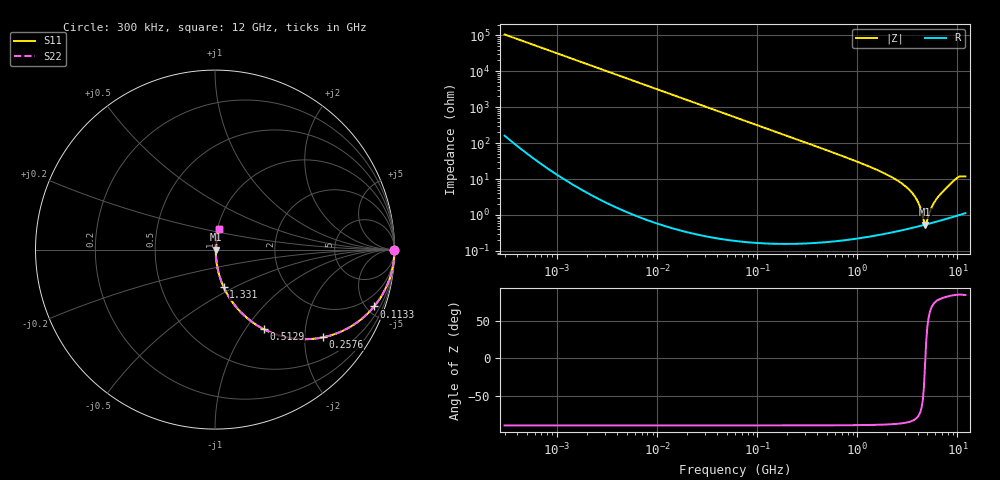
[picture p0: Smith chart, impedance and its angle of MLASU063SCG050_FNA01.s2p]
! MLASU063SCG050_FNA01  S-PARAMETER MODEL  ( Standard Model )
! Model Generated by TAIYO YUDEN Corporation (http://www.ty-top.com)
! Version 1.0
! TAIYO YUDEN Control No. 240819
! Copyright(c) 2024 TAIYO YUDEN CO.,LTD. All Rights Reserved.
! Product Description (link to TY-COMPAS)
! https://ds.yuden.co.jp/TYCOMPAS/or/detail?pn=MLASU063SCG050CFNA01&u=M
! Products Name : Multilayer Ceramic Capacitors
! Characteristics :
!  Capacitance : 5 [pF] , Rated Voltage : 50 [V] , TCC : CG / C0G
!  Case Size : 0.6 x 0.3 / 0.024 x 0.012 [mm/inch] , Thickness : 0.3 / 0.012 [mm/inch]
!  (Conditions: Temperature = 25 [degC] , DC Bias Voltage = 0 [V])
! External Node Assignments :
!  1  o---| |---o  2
! GND o---------o GND
! Frequency Range : 0.3MHz  -  12000MHz  [ 401 STEP ]
# MHZ S RI R 50
! Freq[MHz].  S11 Real  S11 Imag  S21 Real  S21 Imag  S12 Real  S12 Imag  S22 Real  S22 Imag
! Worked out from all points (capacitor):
!   401 points, 300 kHz to 12 GHz, reference 50 ohm
!   read as one part in series: C = 5.01 pF near 316.3 kHz
!   lowest |Z| = 541 mohm at 4.748 GHz (marker M1)
!   series resonance near 4.779 GHz, so ESL is about 220 pH
!   S11 on the Smith chart (normalised r, x): 300 kHz: open; 113.3 MHz: 1.00, -5.60; 257.6 MHz: 1.00, -2.46; 512.9 MHz: 1.00, -1.22; 1.331 GHz: 1.01, -0.44; 12 GHz: 1.02, +0.24
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0.3  1 -0.000945  2.33e-06 0.000945  2.33e-06 0.000945  1 -0.000945
1.769972  1 -0.00558  3.26e-05 0.00558  3.26e-05 0.00558  1 -0.00558
10.44266  0.9989 -0.0329  0.00109 0.0329  0.00109 0.0329  0.9989 -0.0329
60  0.9654 -0.1825  0.0346 0.1825  0.0346 0.1825  0.9654 -0.1825
113.3117  0.8867 -0.3166  0.1133 0.3166  0.1133 0.3166  0.8867 -0.3166
168.5979  0.7793 -0.4143  0.2207 0.4143  0.2207 0.4143  0.7793 -0.4143
257.5933  0.6014 -0.489  0.3986 0.489  0.3986 0.489  0.6014 -0.489
353.9943  0.4431 -0.4958  0.5569 0.4958  0.5569 0.4958  0.4431 -0.4958
512.9422  0.2729 -0.444  0.7271 0.444  0.7271 0.444  0.2729 -0.444
804.7407  0.1294 -0.333  0.8706 0.333  0.8706 0.333  0.1294 -0.333
1331.232  0.0483 -0.2088  0.9517 0.2088  0.9517 0.2088  0.0483 -0.2088
2088.533  0.0179 -0.1203  0.9821 0.1203  0.9821 0.1203  0.0179 -0.1203
2870.14  0.00871 -0.0697  0.9913 0.0697  0.9913 0.0697  0.00871 -0.0697
3547.679  0.00594 -0.0397  0.9941 0.0397  0.9941 0.0397  0.00594 -0.0397
4050.141  0.00524 -0.0217  0.9948 0.0217  0.9948 0.0217  0.00524 -0.0217
4623.766  0.00525 -0.00421  0.9948 0.00421  0.9948 0.00421  0.00525 -0.00421
4747.894  0.00533 -0.00073  0.9947 0.00073  0.9947 0.00073  0.00533 -0.00073
5006.236  0.00556 0.00504  0.9944 -0.00504  0.9944 -0.00504  0.00556 0.00504
5868.704  0.00669 0.0215  0.9933 -0.0215  0.9933 -0.0215  0.00669 0.0215
6879.757  0.00855 0.0388  0.9915 -0.0388  0.9915 -0.0388  0.00855 0.0388
9968.853  0.0207 0.1047  0.9793 -0.1047  0.9793 -0.1047  0.0207 0.1047
12000  0.0243 0.1135  0.9757 -0.1135  0.9757 -0.1135  0.0243 0.1135
